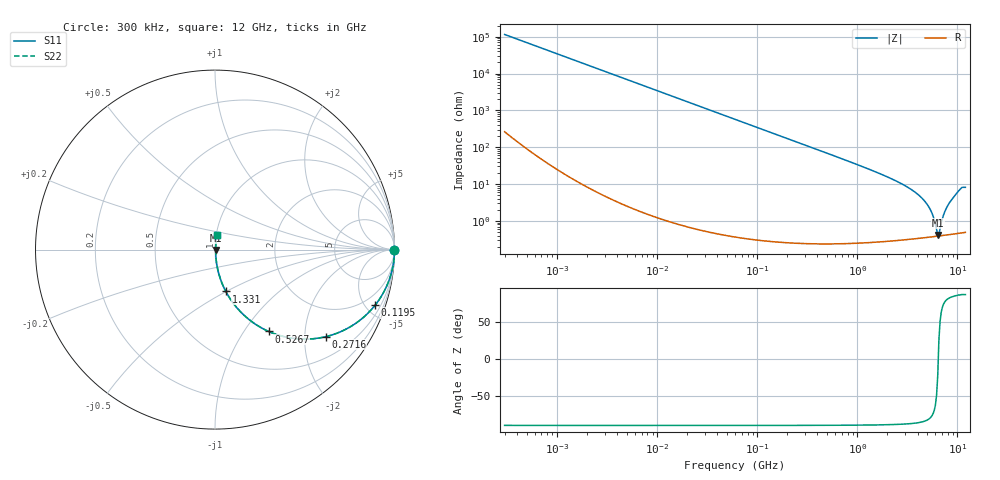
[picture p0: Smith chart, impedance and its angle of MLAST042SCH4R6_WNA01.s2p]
! MLAST042SCH4R6_WNA01  S-PARAMETER MODEL  ( General Type )
! Model Generated by TAIYO YUDEN Corporation (http://www.ty-top.com)
! Version 1.0
! TAIYO YUDEN Control No. 150820
! Copyright(c) 2015 TAIYO YUDEN CO.,LTD. All Rights Reserved.
! Product Description (link to TY-COMPAS)
! https://ds.yuden.co.jp/TYCOMPAS/or/detail?pn=MLAST042SCH4R6BWNA01&u=M
! Products Name : Multilayer Ceramic Capacitors
! Characteristics :
!  Capacitance : 4.6 pF , Rated Voltage : 25V , TCC : CH / C0H
!  Case Size : 0.4 x 0.2 / 0.016 x 0.008 [mm/inch] , Thickness : 0.2 / 0.008 [mm/inch]
!  (Conditions: Temperature = 25 degC , DC Bias Current/Voltage = 0A / 0V)
! External Node Assignments :
!  1  o---| |---o  2
! GND o---------o GND
! Frequency Range : 0.3MHz  -  12000MHz  [ 401 STEP ]
# MHz S RI R 50
! Freq[MHz].  S11 Real  S11 Imag  S21 Real  S21 Imag  S12 Real  S12 Imag  S22 Real  S22 Imag
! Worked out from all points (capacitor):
!   401 points, 300 kHz to 12 GHz, reference 50 ohm
!   read as one part in series: C = 4.61 pF near 316.3 kHz
!   lowest |Z| = 418 mohm at 6.354 GHz (marker M1)
!   series resonance near 6.434 GHz, so ESL is about 130 pH
!   S11 on the Smith chart (normalised r, x): 300 kHz: open; 119.5 MHz: 1.01, -5.78; 271.6 MHz: 1.00, -2.54; 526.7 MHz: 1.00, -1.30; 1.331 GHz: 1.01, -0.50; 12 GHz: 1.01, +0.16
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0.3  1 -0.000868  2.74e-06 0.000868  2.74e-06 0.000868  1 -0.000868
1.769972  1 -0.00512  2.88e-05 0.00512  2.88e-05 0.00512  1 -0.00512
10.44266  0.9991 -0.0302  0.000923 0.0302  0.000923 0.0302  0.9991 -0.0302
60  0.9706 -0.1685  0.0294 0.1685  0.0294 0.1685  0.9706 -0.1685
119.4772  0.8929 -0.3087  0.1071 0.3087  0.1071 0.3087  0.8929 -0.3087
271.6094  0.6171 -0.4851  0.3829 0.4851  0.3829 0.4851  0.6171 -0.4851
353.9943  0.4865 -0.4986  0.5135 0.4986  0.5135 0.4986  0.4865 -0.4986
526.7124  0.2988 -0.4559  0.7012 0.4559  0.7012 0.4559  0.2988 -0.4559
826.3444  0.1462 -0.3503  0.8538 0.3503  0.8538 0.3503  0.1462 -0.3503
1331.232  0.0603 -0.2329  0.9397 0.2329  0.9397 0.2329  0.0603 -0.2329
2088.533  0.0241 -0.1441  0.9759 0.1441  0.9759 0.1441  0.0241 -0.1441
3364.605  0.00866 -0.0738  0.9913 0.0738  0.9913 0.0738  0.00866 -0.0738
4502.883  0.00497 -0.039  0.995 0.039  0.995 0.039  0.00497 -0.039
5420.343  0.00399 -0.0185  0.996 0.0185  0.996 0.0185  0.00399 -0.0185
5715.274  0.00388 -0.0128  0.9961 0.0128  0.9961 0.0128  0.00388 -0.0128
6188.031  0.00383 -0.00435  0.9962 0.00435  0.9962 0.00435  0.00383 -0.00435
6354.153  0.00385 -0.00159  0.9962 0.00159  0.9962 0.00159  0.00385 -0.00159
6699.894  0.00394 0.00464  0.9961 -0.00464  0.9961 -0.00464  0.00394 0.00464
7448.838  0.00435 0.0169  0.9956 -0.0169  0.9956 -0.0169  0.00435 0.0169
8281.503  0.00513 0.03  0.9949 -0.03  0.9949 -0.03  0.00513 0.03
10511.28  0.00939 0.0688  0.9906 -0.0688  0.9906 -0.0688  0.00939 0.0688
12000  0.0113 0.0801  0.9887 -0.0801  0.9887 -0.0801  0.0113 0.0801
